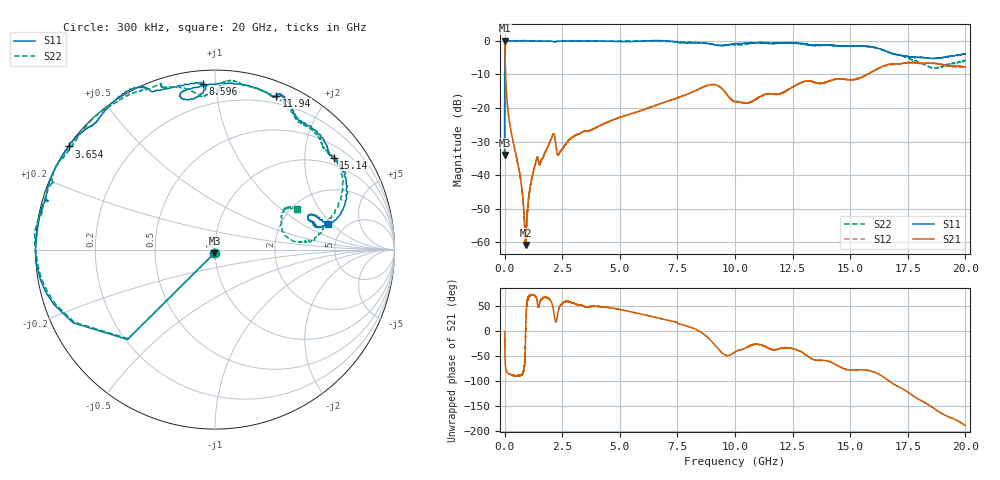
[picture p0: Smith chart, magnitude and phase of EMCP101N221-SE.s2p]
!EMCP101N221
!Johanson Technology Inc.
!www.johansontechnology.com
!Test Board Conditions:
!Substrate Type  RO4350B
!Substrate Thickness  10 mil
!Substrate Dk  3.66
!TL Type: GCPW
!TL Trace Width  20 mil
!TL Gap  10 mil
!PART MODE SINGLE ENDED (AKA BYPASS)
!DUT TOPOLOGY	SERIES-SHUNT
# MHz S  dB  R 50
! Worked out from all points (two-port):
!   20001 points, 300 kHz to 20 GHz, reference 50 ohm
!   highest |S21| = 0.01 dB at 300 kHz (marker M1); lowest = -60.8 dB at 909.3 MHz (marker M2)
!   |S21| within 3 dB of the highest: start of sweep to 13.63 MHz
!   lowest |S11| = -34.0 dB at 300 kHz (marker M3), VSWR 1.04, Z = 49.6 - j1.94 ohm
!   |S11| at or under -10 dB: start of sweep to 4.588 MHz
!   |S22| runs from -34.2 to 0.1 dB; largest |S21 - S12| = 0.017
!   S11 on the Smith chart (normalised r, x): 300 kHz: 0.99, -0.04; 3.654 GHz: 0.00, +0.32; 8.596 GHz: 0.07, +0.93; 11.94 GHz: 0.13, +1.47; 15.14 GHz: 0.79, +2.71; 20 GHz: 3.66, +1.78
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0.3  -34.04 -99.7  0.01 -1.2  -0.00 -1.5  -34.25 -96.4
111.298  -0.04 -174.2  -18.41 -83.4  -18.37 -83.4  -0.12 -173.6
246.296  0.00 -179.3  -25.77 -87.4  -25.72 -87.7  -0.03 -178.3
687.29  -0.03 174.1  -40.93 -89.2  -40.90 -88.7  0.06 176.6
909.286  -0.05 171.7  -60.84 -10.3  -60.16 -10.7  0.07 174.3
1137.283  -0.04 169.4  -42.45 72.1  -42.50 73.2  0.04 171.9
1375.279  -0.06 167.1  -35.61 66.0  -35.56 66.6  -0.05 169.2
2086.269  -0.19 163.8  -28.07 50.0  -28.03 49.9  -0.17 157.7
2359.265  -0.11 162.6  -33.69 45.4  -33.66 44.9  -0.07 156.2
3334.25  -0.01 149.0  -27.34 51.5  -27.35 51.5  -0.02 149.9
3654.245  -0.02 144.8  -26.83 48.4  -26.83 48.4  -0.08 149.0
6667.2  0.08 118.0  -18.97 25.8  -18.91 25.5  -0.12 119.4
8596.171  -0.65 94.2  -13.84 -4.8  -13.87 -5.1  -0.58 104.7
9224.162  -1.35 96.5  -13.29 -33.5  -13.31 -32.8  -1.25 96.1
10000.15  -0.90 100.9  -18.12 -42.2  -17.93 -42.0  -1.13 90.2
11207.13  -0.67 73.6  -16.19 -29.4  -16.37 -29.4  -0.48 83.9
11943.12  -0.70 68.3  -15.82 -35.6  -15.73 -34.6  -0.62 77.8
13334.1  -1.29 58.4  -12.11 -56.1  -12.09 -56.5  -1.37 58.1
15139.07  -1.55 37.8  -11.59 -78.3  -11.41 -77.1  -1.55 39.0
16667.05  -3.42 13.2  -7.01 -99.7  -7.21 -99.3  -3.36 16.4
18535.02  -5.26 18.1  -6.69 -152.2  -6.57 -153.0  -8.03 12.3
20000  -3.85 12.9  -7.82 170.4  -7.96 172.1  -5.84 26.7
